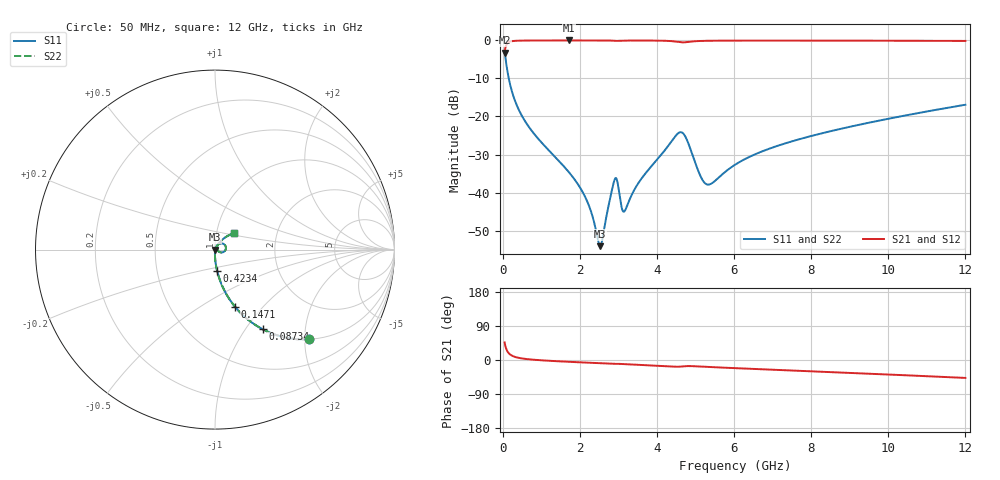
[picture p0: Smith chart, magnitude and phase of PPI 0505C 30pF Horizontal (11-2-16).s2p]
# MHz S MA R 50
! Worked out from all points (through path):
!   1601 points, 50 MHz to 12 GHz, reference 50 ohm
!   highest |S21| = -0.01 dB at 1.723 GHz (marker M1); lowest = -3.3 dB at 50 MHz (marker M2)
!   group delay of S21, straight-line fit = 12 ps
!   lowest |S11| = -54.1 dB at 2.53 GHz (marker M3), VSWR 1.00, Z = 50.2 - j0.047 ohm
!   |S11| at or under -10 dB: 157.8 MHz to end of sweep
!   |S22| runs from -54.1 to -2.8 dB; largest |S21 - S12| = 0
!   S11 on the Smith chart (normalised r, x): 50 MHz: 0.99, -2.10; 87.34 MHz: 0.99, -1.20; 147.1 MHz: 0.99, -0.71; 423.4 MHz: 1.00, -0.24; 12 GHz: 1.22, +0.23
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50  0.7258 -43.6  0.6876 46.4  0.6876 46.4  0.7258 -43.6
87.34375  0.5168 -59.1  0.8558 30.8  0.8558 30.8  0.5168 -59.1
147.0938  0.3369 -70.7  0.9411 19.2  0.9411 19.2  0.3369 -70.7
423.4375  0.1209 -84.2  0.992 5.5  0.992 5.5  0.1209 -84.2
819.2812  0.05877 -88.5  0.9973 0.6  0.9973 0.6  0.05877 -88.5
1723  0.01838 -90.8  0.9984 -4.8  0.9984 -4.8  0.01838 -90.8
2044.156  0.0108 -88.7  0.9984 -6.3  0.9984 -6.3  0.0108 -88.7
2260.75  0.00625 -82.7  0.9983 -7.3  0.9983 -7.3  0.00625 -82.7
2529.625  0.001973 -13.7  0.9979 -8.6  0.9979 -8.6  0.001973 -13.7
2910.531  0.01511 26.0  0.9876 -10.4  0.9876 -10.4  0.01511 26.0
2962.812  0.01464 3.7  0.9856 -10.2  0.9856 -10.2  0.01464 3.7
3157  0.005659 27.7  0.9954 -10.9  0.9954 -10.9  0.005659 27.7
3515.5  0.01324 63.5  0.9965 -12.6  0.9965 -12.6  0.01324 63.5
4038.312  0.02834 61.7  0.9929 -15.2  0.9929 -15.2  0.02834 61.7
4620.875  0.06218 13.6  0.9459 -17.4  0.9459 -17.4  0.06218 13.6
4755.312  0.05219 -12.1  0.9476 -16.2  0.9476 -16.2  0.05219 -12.1
5113.812  0.01714 -19.3  0.9825 -17.2  0.9825 -17.2  0.01714 -19.3
5278.125  0.01292 4.7  0.9877 -18.0  0.9877 -18.0  0.01292 4.7
6025  0.02318 54.7  0.9938 -21.5  0.9938 -21.5  0.02318 54.7
8019.156  0.05567 56.0  0.994 -29.9  0.994 -29.9  0.05567 56.0
10013.31  0.09359 49.1  0.9908 -38.4  0.9908 -38.4  0.09359 49.1
12000  0.1427 40.8  0.9844 -47.3  0.9844 -47.3  0.1427 40.8
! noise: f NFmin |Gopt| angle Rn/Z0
50  0.0003898  0.8654  0.807  0.0006218
1372  0.003995  0.6748  4.788  0.002365
2701  0.008859  0.7067  9.137  0.005898
4031  0.01597  0.7519  13.55  0.01281
5360  0.02347  0.7742  18.01  0.02072
6682  0.01733  0.6486  22.18  0.009027
8012  0.01798  0.6079  26.26  0.008077
9341  0.01958  0.5896  30.23  0.008179
1.067e+04  0.02152  0.5811  34.09  0.008604
1.2e+04  0.02367  0.5784  37.83  0.009207
